PROGRAM MAIN
VAR
 	myState : E_State;
	nDBID: INT := 4; // referencing id of the nosql database
	sNetID : STRING := '';
		
	fbNoSQLQueryBuilder_DocumentDB: FB_NoSQLQueryBuilder_DocumentDB;
    InsertQueryOptions: T_QueryOptionDocumentDB_Insert;
    sDocument : STRING(2000);
	
	fbNoSQLQuery: FB_NoSQLQueryEvt(sNetID := sNetID, tTimeout := TIME#15S0MS);
    fbJsonDataType: FB_JsonReadWriteDatatype;
	
	
	AggregationQueryOptions: T_QueryOptionDocumentDB_Aggregate;
    sPipeStages: STRING(1000);
	
    fbNoSQLResult: FB_NoSQLResultEvt(sNetID := sNetID, tTimeout := TIME#15S0MS);	 
    aRdStruct : ARRAY [0..9] OF ST_MainStructure;
	
	fbNoSqlValidation : FB_NoSQLValidationEvt(sNetID := sNetID, tTimeout := TIME#15S0MS);
    aIssues : ARRAY[0..99] OF STRING(512);
    aRemaining : ARRAY [0..9] OF STRING(1000);
	
	InfoResult: I_TcMessage;

END_VAR

CASE myState OF
			
	E_State.idle:
		;
		
		
	E_State.init: // init all values and functionsblocks
	
		InsertQueryOptions.pDocuments:= ADR(sDocument); 
		InsertQueryOptions.cbDocuments:= SIZEOF(sDocument);
		fbNoSQLQueryBuilder_DocumentDB.eQueryType := E_DocumentDbQueryType.InsertOne;
		fbNoSQLQueryBuilder_DocumentDB.sCollectionName := 'myCollection';
		fbNoSQLQueryBuilder_DocumentDB.pQueryOptions := ADR(InsertQueryOptions);
		fbNoSQLQueryBuilder_DocumentDB.cbQueryOptions := SIZEOF(InsertQueryOptions);
		
		myState := E_State.write;
		
		
	E_State.write: 
		// write values to the nosql database		
		 
		// set datatypes directly (e.g. MongoDB)
		// sDocument := '{…"myTimestamp": ISODate("2019-02-01T14:46:06.0000000"), …}';
		
		// set the document by JsonDataType
		// sTypeName := fbJsonDataType.GetDatatypeNameByAddress(SIZEOF(anyValue[1]), ADR(anyValue[1]));
		// sDocument := fbJsonDataType.GetJsonStringFromSymbol(sTypeName, SIZEOF(anyValue [1]), ADR(anyValue [1])); 
		
		// set the document yourself as json format (Example)
        sDocument := 
			'{"myBool" : true, 
              "Name" : "Some Name Value",
              "Value": 2.3,
              "Value2":3, 
              "Child":{"Name":"Single Child", 
                       "Value":1, 
                       "myBool":true, 
                       "arr":[12.0,13.0,14.0,15.0], 
                       "myBool2" : true}, 
              "Children":[
                       {"Name":"Child1"
                       ,"Value": 1, 
                       "myBool" : true, 
                       "arr":[12.1,13.1,14.1,15.1], 
                       "myBool2" : true},
                       {"Name":"Child2",
                       "Value":2, 
                       "myBool" : true, 
                       "arr":[12.2,13.2,14.2,15.2], 
                       "myBool2" : true},
                       {"Name":"Child3",
                       "Value":1, 
                       "myBool" : true, 
                       "arr":[12.3,13.3,14.3,15.3], 
                       "myBool2" : true}]
			  }';
			  
		IF fbNoSQLQuery.Execute(nDBID, fbNoSQLQueryBuilder_DocumentDB) THEN
            IF fbNoSQLQuery.bError THEN
                InfoResult := fbNoSQLQuery.ipTcResult;
                myState:= E_State.error;
            ELSE
                myState:= E_State.idle; 
            END_IF
        END_IF
		
		
	E_State.aggregation: // aggregation of nosql data
	
		AggregationQueryOptions.pPipeStages := ADR(sPipeStages);
		AggregationQueryOptions.cbPipeStages := SIZEOF(sPipeStages);
		fbNoSQLQueryBuilder_DocumentDB.eQueryType := E_DocumentDbQueryType.Aggregation;
		fbNoSQLQueryBuilder_DocumentDB.sCollectionName := 'myCollection';
		fbNoSQLQueryBuilder_DocumentDB.pQueryOptions := ADR(AggregationQueryOptions);
		fbNoSQLQueryBuilder_DocumentDB.cbQueryOptions := SIZEOF(AggregationQueryOptions);
		
		// set pipeline stages for aggregation:
		sPipeStages :='{$$match :{}}';
		
        IF fbNoSQLQuery.ExecuteDataReturn(nDBID, fbNoSQLQueryBuilder_DocumentDB, pNoSqlResult:= ADR(fbNoSQLResult)) THEN
            IF fbNoSQLQuery.bError THEN
                InfoResult := fbNoSQLQuery.ipTcResult;
                myState:= E_State.error;
            ELSE
                myState:= E_State.readstruct; 
            END_IF
        END_IF
		
		
	E_State.readstruct: // read the data to the destination structure
	
		IF fbNoSQLResult.ReadAsStruct(0, 4, ADR(aRdStruct), SIZEOF(aRdStruct), bValidate := TRUE, ADR(fbNoSqlValidation), bDataRelease:= TRUE) THEN
            IF fbNoSQLResult.bError THEN
                InfoResult := fbNoSQLResult.ipTcResult;
                myState:= E_State.error;
            ELSE
                myState:= E_State.idle; 
            END_IF
        END_IF
		
		
	E_State.validationIssues: // read the validation issues from the validation as string array
	
		IF fbNoSqlValidation.GetIssues(ADR(aIssues), SIZEOF(aIssues), FALSE) THEN
            IF fbNoSqlValidation.bError THEN
                InfoResult := fbNoSqlValidation.ipTcResult;
                 myState:= E_State.error;
            ELSE
                myState:= E_State.idle; 
            END_IF
	    END_IF
		
		
	E_State.validationRemaining: // validate remaining data that could not be copied to the results
	
		IF fbNoSqlValidation.GetRemainingData(ADR(aRemaining), SIZEOF(aRemaining), SIZEOF(aRemaining[1]), bDataRelease:= FALSE)THEN
            IF fbNoSqlValidation.bError THEN
                InfoResult := fbNoSqlValidation.ipTcResult;
                myState:= E_State.error;
            ELSE
                myState:= E_State.idle; 
            END_IF
		END_IF
		
	E_State.error: // error handling
		;
	
	
	
	
	
	
	

	
END_CASE

END_PROGRAM
